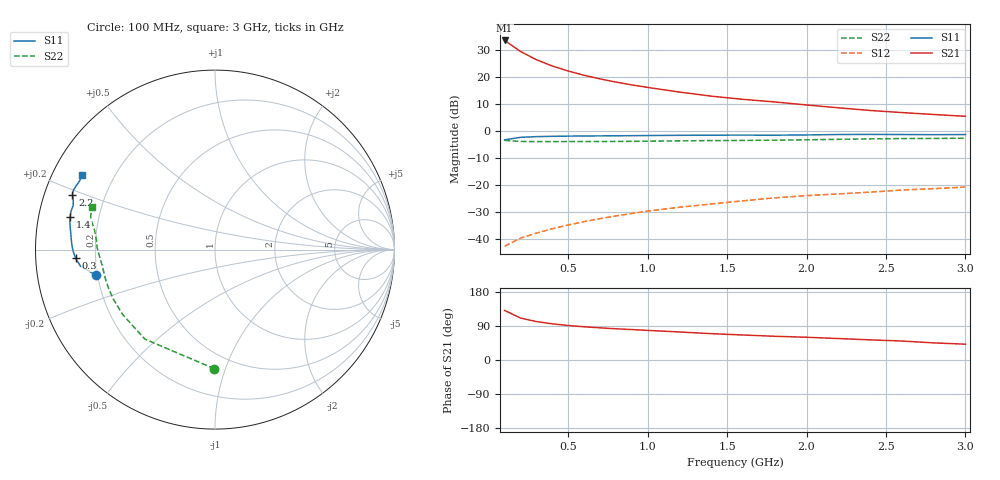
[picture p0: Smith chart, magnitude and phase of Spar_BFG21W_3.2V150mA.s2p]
! Filename: 3_2150bfg21.001
! Title: BFG21W
! Bias: Vce=3.2V; Ic=150mA
! Company: NXP Semiconductors NL
! User: Quality&Reliability T&D
! Measure time: 10 Nov 1999 / 11:43:19
#  MHz  S  MA  R 50
! Freq  S11  S21  S12  S22  :
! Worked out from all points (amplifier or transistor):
!   20 points, 100 MHz to 3 GHz, reference 50 ohm
!   highest |S21| = 33.4 dB at 100 MHz (marker M1)
!   |S21| within 3 dB of that: start of sweep to 173.6 MHz
!   unconditionally stable (mu >= 1): 591.2 MHz to end of sweep
!   at 400 MHz: K = 0.93, MSG = 30.1 dB, |S12| = -36.3 dB
!   at 1.2 GHz: K = 1.06, MAG = 19.9 dB, |S12| = -28.3 dB
!   at 3 GHz: K = 1.05, MAG = 11.7 dB, |S12| = -20.9 dB
!   S11 on the Smith chart (normalised r, x): 100 MHz: 0.19, -0.10; 300 MHz: 0.13, -0.03; 1.4 GHz: 0.10, +0.11; 2.2 GHz: 0.08, +0.18; 3 GHz: 0.09, +0.26
100  0.6787 -167.9  46.93 130.7  0.007293 59.4  0.6635 -90.4
200  0.7553 -173.0  29.35 110.7  0.01026 56.9  0.6337 -128.1
300  0.7779 -176.4  20.64 101.4  0.01273 59.8  0.6289 -144.9
400  0.7885 -178.9  15.8 95.5  0.01532 63.5  0.6303 -154.2
500  0.7951 179.2  12.75 91.1  0.01798 66.0  0.6312 -160.1
600  0.7992 177.5  10.64 87.7  0.02074 68.0  0.6318 -164.3
700  0.8029 176.0  9.129 84.9  0.02358 69.8  0.6319 -167.6
800  0.806 174.5  7.968 82.4  0.02646 71.0  0.6333 -170.3
900  0.8101 173.0  7.066 80.3  0.0294 72.4  0.6362 -172.7
1000  0.8147 171.7  6.345 78.1  0.03251 72.9  0.64 -174.9
1200  0.8231 169.2  5.204 74.0  0.03831 73.4  0.6492 -178.3
1400  0.8281 167.2  4.369 69.5  0.04398 73.4  0.6572 178.9
1600  0.83 165.1  3.813 66.0  0.05038 73.4  0.6611 176.3
1800  0.8274 162.7  3.413 62.6  0.05724 73.2  0.6684 173.6
2000  0.836 160.8  3.002 60.0  0.06284 73.6  0.68 170.9
2200  0.851 158.9  2.66 56.6  0.0677 73.1  0.6938 168.6
2400  0.8554 157.2  2.372 53.2  0.07301 72.2  0.7075 166.9
2600  0.8513 155.3  2.171 50.1  0.0798 71.0  0.7163 165.4
2800  0.8456 153.0  1.999 45.2  0.08474 69.2  0.7199 163.4
3000  0.8497 150.5  1.85 41.7  0.09056 68.2  0.7264 160.9
